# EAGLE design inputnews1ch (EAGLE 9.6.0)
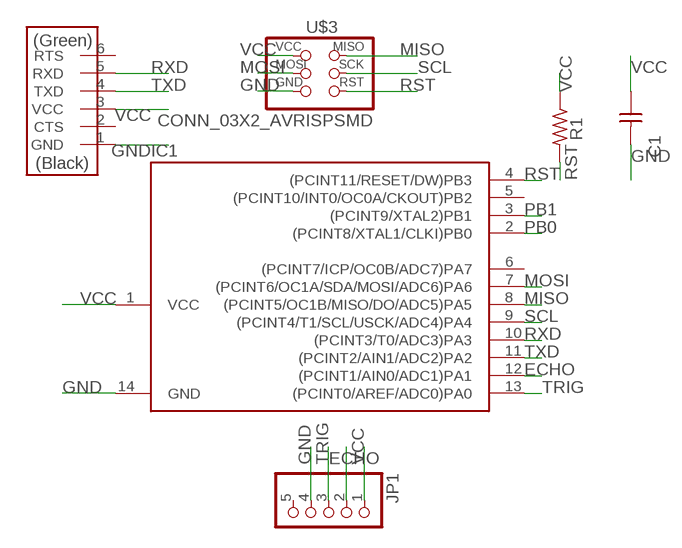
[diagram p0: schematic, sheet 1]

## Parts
C1  CAP_UNPOLARIZEDFAB  [C1206FAB]
IC1  UC_ATTINY44-SSU  [SOIC14]
JP1  PINHD-1X5  [1X05]
R1  R1206FAB  [R1206FAB]
U$2  CONN_06_FTDI-SMD-HEADER  [1X06SMD]
U$3  CONN_03X2_AVRISPSMD  [2X03SMD]

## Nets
ECHO: IC1.12((PCINT1/AIN0/ADC1)PA1) JP1.2
GND: C1.2 IC1.14(GND) JP1.4 U$2.1(GND) U$3.6(GND)
MISO: IC1.8((PCINT5/OC1B/MISO/DO/ADC5)PA5) U$3.1(MISO)
MOSI: IC1.7((PCINT6/OC1A/SDA/MOSI/ADC6)PA6) U$3.4(MOSI)
PB0: IC1.2((PCINT8/XTAL1/CLKI)PB0)
PB1: IC1.3((PCINT9/XTAL2)PB1)
RST: IC1.4((PCINT11/RESET/DW)PB3) R1.2 U$3.5(RST)
RXD: IC1.10((PCINT3/T0/ADC3)PA3) U$2.5(RXD)
SCL: IC1.9((PCINT4/T1/SCL/USCK/ADC4)PA4) U$3.3(SCK)
TRIG: IC1.13((PCINT0/AREF/ADC0)PA0) JP1.3
TXD: IC1.11((PCINT2/AIN1/ADC2)PA2) U$2.4(TXD)
VCC: C1.1 IC1.1(VCC) JP1.1 R1.1 U$2.3(VCC) U$3.2(VCC)
Unconnected: IC1.5((PCINT10/INT0/OC0A/CKOUT)PB2) IC1.6((PCINT7/ICP/OC0B/ADC7)PA7) JP1.5 U$2.2(CTS) U$2.6(RTS)

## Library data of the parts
C1 = fab:CAP_UNPOLARIZED
IC1 = fab:UC_ATTINY44
JP1 = pinhead:PINHD-1X5: PIN HEADER
R1 = fab:R: Resistor (US Symbol)
U$2 = fab:CONN_06_FTDI-SMD-HEADER
U$3 = fab:CONN_03X2_AVRISP

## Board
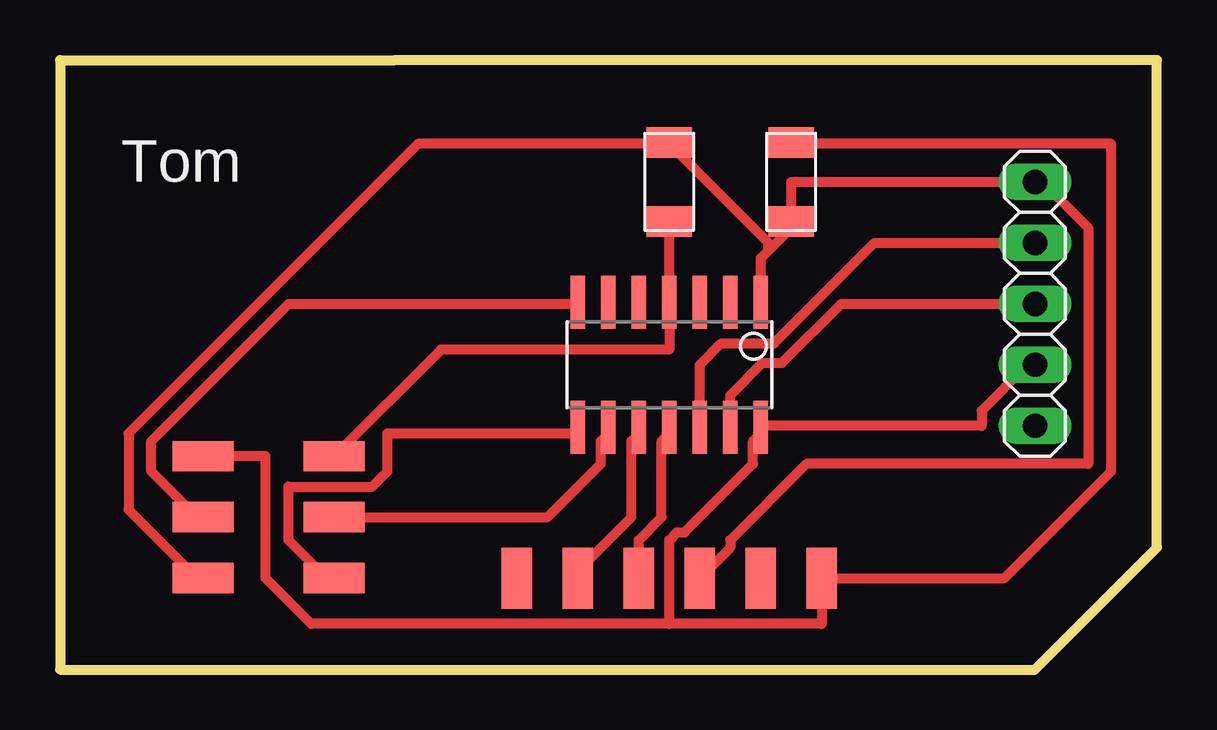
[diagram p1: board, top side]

Size 45.72 x 25.4 mm. Coordinates in mm from the lower left corner, seen from the top.
Outline: 0,25.4 0,0 40.64,0 45.72,5.08 45.72,25.4 15.24,25.4 13.97,25.4 0,25.4
Copper layers (1*16): Top 0.035mm / dielectric 1.5mm / Bottom 0.035mm
Design rules "default *": minimum track width 16mil, minimum drill 0.35mm, track to track 16mil, track to pad 16mil, pad to pad 16mil, via to via 16mil, smd to smd 16mil, copper to edge 40mil, drill to drill 6mil, minimum pad ring 10mil, minimum via ring 8mil, stop-mask expansion 4mil, vias tented up to drill 0mil, thermal gap 10mil

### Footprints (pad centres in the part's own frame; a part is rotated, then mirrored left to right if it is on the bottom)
C1206FAB = smd 1.27 x 1.905: 1 -1.651,0; 2 1.651,0
SOIC14 = smd 0.61 x 2.21: 1 -3.81,-2.603; 2 -2.54,-2.603; 3 -1.27,-2.603; 4 0,-2.603; 5 1.27,-2.603; 6 2.54,-2.603; 7 3.81,-2.603; 8 3.81,2.603; 9 2.54,2.603; 10 1.27,2.603; 11 0,2.603; 12 -1.27,2.603; 13 -2.54,2.603; 14 -3.81,2.603
1X05 = drill 1.016 long: 1 -5.08,0; 2 -2.54,0; 3 0,0; 4 2.54,0; 5 5.08,0
R1206FAB = smd 1.27 x 1.905: 1 -1.651,0; 2 1.651,0
1X06SMD = smd 2.54 x 1.27: 1 0,6.35; 2 0,3.81; 3 0,1.27; 4 0,-1.27; 5 0,-3.81; 6 0,-6.35
2X03SMD = smd 2.54 x 1.27: 1 -2.54,2.54; 2 2.92,2.54; 3 -2.54,0; 4 2.92,0; 5 -2.54,-2.54; 6 2.92,-2.54

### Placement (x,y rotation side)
C1  30.48,20.32 90 top
IC1  25.4,12.7 180 top
JP1  40.64,15.24 270 top
R1  25.4,20.32 270 top
U$2  25.4,3.81 270 top
U$3  8.89,6.35 180 top

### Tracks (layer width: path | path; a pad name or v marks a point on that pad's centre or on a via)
ECHO
  Top 0.406: IC1.12 26.67,12.7 27.56,13.59 29.77,13.59 33.96,17.78 JP1.2
GND
  Top 0.406: JP1.4 40.32,12.7 38.42,10.79 38.42,10.16 29.21,10.16 IC1.14 29.21,9.84 28.89,9.53 28.89,8.57 26.04,5.71 25.72,5.71 25.4,5.4 25.4,1.91 | C1.2 30.48,21.91 43.81,21.91 43.81,8.26 39.37,3.81 U$2.1 31.75,1.91 25.4,1.91 | U$3.6 8.57,8.89 8.57,3.81 10.48,1.91 25.4,1.91
MISO
  Top 0.406: U$3.1 11.11,3.81 9.52,5.4 9.52,7.62 13.02,7.62 13.65,8.26 13.65,9.84 21.59,9.84 IC1.8
MOSI
  Top 0.406: IC1.7 21.59,15.24 9.52,15.24 3.81,9.53 3.81,8.26 5.72,6.35 U$3.4
RST
  Top 0.406: R1.2 IC1.4 25.4,13.34 15.88,13.34 U$3.5
RXD
  Top 0.406: U$2.5 21.59,4.13 23.81,6.35 23.81,9.53 24.13,9.84 IC1.10
SCL
  Top 0.406: U$3.3 20.32,6.35 22.54,8.57 22.54,9.53 22.86,9.84 IC1.9
TRIG
  Top 0.406: 27.94,10.16 IC1.13 27.94,11.43 29.29,12.78 30.1,12.78 32.57,15.24 JP1.3
TXD
  Top 0.406: U$2.4 24.13,5.4 25.08,6.35 25.08,9.53 25.4,9.84 IC1.11
VCC
  Top 0.406: U$2.3 27.94,5.08 27.94,5.4 31.12,8.57 42.86,8.57 42.86,18.41 40.96,20.32 JP1.1 30.48,20.32 C1.1 30.48,18.41 29.53,17.46 | 29.53,17.46 29.21,17.14 IC1.1 | 25.4,21.91 29.53,17.78 29.53,17.46 | 25.4,21.91 14.92,21.91 2.86,9.84 2.86,6.67 5.72,3.81 U$3.2 | 25.4,21.91 R1.1

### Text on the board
tNames: Tom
